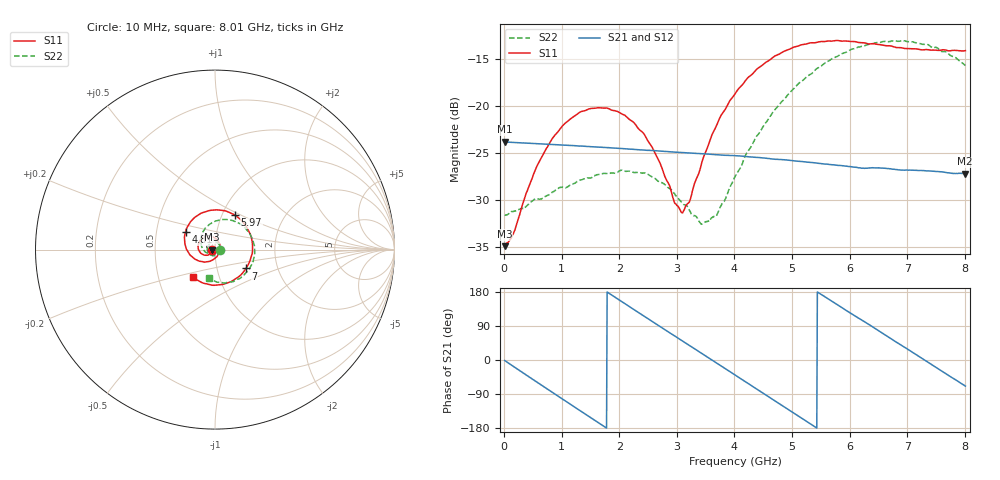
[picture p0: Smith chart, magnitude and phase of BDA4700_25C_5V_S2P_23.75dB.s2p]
!Agilent Technologies,E5071B,MY42404982,A.09.10
!Date: Mon Oct 20 13:38:23 2025
!Data & Calibration Information:
!Freq	S11:SOLT2(ON)	S21:SOLT2(ON)	S12:SOLT2(ON)	S22:SOLT2(ON)
# Hz S RI R 50
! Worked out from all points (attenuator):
!   801 points, 10 MHz to 8.01 GHz, reference 50 ohm
!   highest |S21| = -23.83 dB at 10 MHz (marker M1); lowest = -27.2 dB at 8 GHz (marker M2)
!   lowest |S11| = -35.0 dB at 10 MHz (marker M3), VSWR 1.04, Z = 48.2 - j0.0993 ohm
!   |S11| at or under -10 dB: start of sweep to end of sweep
!   |S22| runs from -32.6 to -13.0 dB; largest |S21 - S12| = 0.00048
!   S11 on the Smith chart (normalised r, x): 10 MHz: 0.96, -0.00; 4.81 GHz: 0.71, +0.14; 5.97 GHz: 1.15, +0.46; 7 GHz: 1.38, -0.30; 8.01 GHz: 0.75, -0.24
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1e7  -0.0179 -0.00103  0.0644 -0.00138  0.0643 -0.00142  0.0261 -0.000835
1.6e8  -0.0186 -0.00928  0.0611 -0.0183  0.0612 -0.0183  0.0263 -0.0075
5.3e8  -0.0345 -0.0283  0.0369 -0.0511  0.0368 -0.0512  0.0162 -0.0275
7.7e8  -0.0532 -0.0315  0.0125 -0.0612  0.0126 -0.0612  0.00104 -0.0335
1.35e9  -0.0935 0.00411  -0.0445 -0.0419  -0.0445 -0.0419  -0.0363 -0.0177
2.09e9  -0.0521 0.0726  -0.051 0.03  -0.051 0.0301  -0.029 0.0344
2.42e9  -0.0106 0.0708  -0.0262 0.0519  -0.0262 0.052  -0.00447 0.0435
2.68e9  0.0159 0.0491  -0.00119 0.0575  -0.00121 0.0575  0.0133 0.0373
2.97e9  0.0281 0.0109  0.026 0.0503  0.026 0.0502  0.0259 0.0213
3.11e9  0.0257 -0.00918  0.0371 0.0425  0.037 0.0425  0.0283 0.0101
3.41e9  0.0013 -0.0466  0.0525 0.0186  0.0526 0.0185  0.0204 -0.0121
3.54e9  -0.0157 -0.0589  0.055 0.00648  0.055 0.00637  0.0128 -0.0207
3.7e9  -0.043 -0.0674  0.0542 -0.00854  0.0542 -0.00873  -0.000977 -0.0265
4.01e9  -0.1 -0.0586  0.0419 -0.0345  0.0419 -0.0345  -0.0327 -0.0259
4.81e9  -0.1639 0.0987  -0.0246 -0.0455  -0.0245 -0.0457  -0.0782 0.0693
5.35e9  -0.0696 0.2057  -0.0493 -0.0073  -0.0494 -0.00748  -0.0153 0.1487
5.97e9  0.1116 0.1909  -0.0293 0.0375  -0.0295 0.0375  0.1251 0.1504
6.68e9  0.2089 -0.00583  0.0233 0.04  0.0234 0.0399  0.2199 -0.00109
7e9  0.1731 -0.1047  0.0397 0.0223  0.0398 0.0221  0.2024 -0.0867
7.5e9  0.0367 -0.1949  0.0422 -0.015  0.0422 -0.0151  0.101 -0.1788
8e9  -0.1191 -0.1565  0.0164 -0.0404  0.0164 -0.0405  -0.0295 -0.1624
8.01e9  -0.1217 -0.1549  0.0157 -0.0407  0.0158 -0.0408  -0.0318 -0.161
